PROGRAM MAIN
VAR
	in_Req          AT%I*  : BOOL   := FALSE;
	
	out_Measure     AT%Q*  : UDINT  := 0;
	out_ProductID   AT%Q*  : UDINT  := 0;
	out_Ack         AT%Q*  : BOOL;
	
	request         : BOOL := FALSE;
	isReady         : BOOL;
	
	FB_R_TRIG       : R_TRIG;
	FB_F_TRIG       : F_TRIG;
	FB_GetMeasure   : GETMEASURE;
	FB_TON          : TON;
END_VAR

(*	START: 	Detecting an incomming request 
			to deliver the measure of the next product*)
	FB_R_TRIG( CLK := in_Req );
	IF FB_R_TRIG.Q THEN
		out_Ack := FALSE;
		request := TRUE;
	END_IF
	
	FB_F_TRIG( 	CLK := in_Req );
	IF FB_F_TRIG.Q THEN
		out_Ack := FALSE;
		request := FALSE;
	END_IF
(*	END: 	Detecting an incomming request*)

(*	START: 	Simulating duration for measuring the next product*)
IF isReady THEN
	IF request THEN 
		FB_GetMeasure(	nominalMeasure := 5000, 
						variance := 1000, 
						steps := 100, 
						measure => out_Measure );
						
		out_ProductID := out_ProductID + 1;
		request := FALSE;	
		isReady := FALSE;
		out_Ack := TRUE;
	END_IF	
ELSE
	FB_TON( PT := T#200MS, 
			IN := NOT FB_TON.Q );
	
	isReady := FB_TON.Q;
END_IF
(*	END: 	Simulating duration for measuring the next product*)

END_PROGRAM
